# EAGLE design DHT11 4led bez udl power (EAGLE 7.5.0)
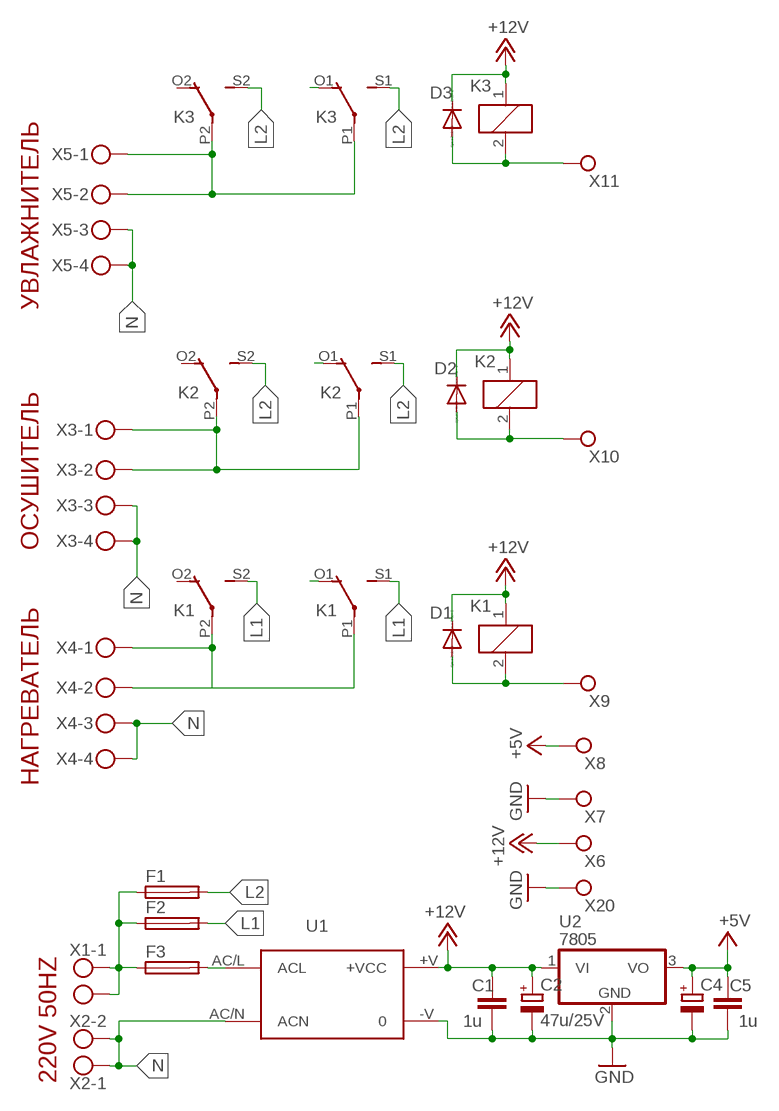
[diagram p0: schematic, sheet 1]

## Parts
C1  1u  C-EUC1206  [C1206]
C2  47u/25V  CPOL-EUE2.5-5  [E2,5-5]
C4  47u/25V  CPOL-EUE2.5-5  [E2,5-5]
C5  1u  C-EUC1206  [C1206]
D1  1N4004  [DO41-10]
D2  1N4004  [DO41-10]
D3  1N4004  [DO41-10]
F1  FUSEGSH15 10A 5x20mm  FUSEGSH15  [GSH15]
F2  FUSEGSH15 10A 5x20mm  FUSEGSH15  [GSH15]
F3  FUSEGSH15 1A 5x20mm  FUSEGSH15  [GSH15]
K1  4052  [F4052]
K2  4052  [F4052]
K3  4052  [F4052]
U1  IRM10-12  [IRM10-12]
U2  7805  7805T  [TO220H]
X1  MKDSN1,5/2-5,08  [MKDSN1,5/2-5,08]
X2  MKDSN1,5/2-5,08  [MKDSN1,5/2-5,08]
X3  MKDSN1,5/4-5,08  [MKDSN1,5/4-5,08]
X4  MKDSN1,5/4-5,08  [MKDSN1,5/4-5,08]
X5  MKDSN1,5/4-5,08  [MKDSN1,5/4-5,08]
X6  TPPAD1-17Y  [P1-17Y]
X7  TPPAD1-17Y  [P1-17Y]
X8  TPPAD1-17Y  [P1-17Y]
X9  TPPAD1-17Y  [P1-17Y]
X10  TPPAD1-17Y  [P1-17Y]
X11  TPPAD1-17Y  [P1-17Y]
X20  TPPAD1-17Y  [P1-17Y]

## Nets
+5V: C4.+ C5.1 U2.3(VO) X8.TP
+12V: C1.1 C2.+ D1.C D2.C D3.C K1.1 K2.1 K3.1 U1.+V(+VCC) U2.1(VI) X6.TP
GND: C1.2 C2.- C4.- C5.2 U1.-V U2.2(GND) X7.TP X20.TP
L1: F2.2 K1.S1(2:S) K1.S2(3:S)
L2: F1.2 K2.S1(2:S) K2.S2(3:S) K3.S1(2:S) K3.S2(3:S)
N: U1.AC/N(ACN) X2.1 X2.2 X3.3 X3.4 X4.3 X4.4 X5.3 X5.4
N$1: D3.A K3.2 X11.TP
N$2: K3.P1(2:P) K3.P2(3:P) X5.1 X5.2
N$3: K3.O1(2:O)
N$28: F1.1 F2.1 F3.1 X1.1 X1.2
N$29: F3.2 U1.AC/L(ACL)
N$41: D2.A K2.2 X10.TP
N$43: K2.P1(2:P) K2.P2(3:P) X3.1 X3.2
N$45: K2.O1(2:O)
N$48: D1.A K1.2 X9.TP
N$52: K1.O1(2:O)
N$53: K1.P1(2:P) K1.P2(3:P) X4.1 X4.2
Unconnected: K1.O2(3:O) K2.O2(3:O) K3.O2(3:O)

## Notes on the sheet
- УВЛАЖНИТЕЛЬ
- ОСУШИТЕЛЬ
- НАГРЕВАТЕЛЬ
- 220V 50HZ

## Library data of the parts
C1 C5 = rcl:C-EU: CAPACITOR, European symbol
C2 C4 = rcl:CPOL-EU: POLARIZED CAPACITOR, European symbol
D1-D3 = diode:1N4004: DIODE
F1-F3 = fuse:FUSE: Fuse; OC_FARNELL: unknown; OC_NEWARK: unknown
K1-K3 = relay:4052: RELAY 2 x switch, Finder; OC_FARNELL: unknown; OC_NEWARK: unknown
U1 = acdc:IRM10-12
U2 = linear:78*: Positive VOLTAGE REGULATOR Source: http://cache.national.com/ds/LM/LM78L05.pdf http://www.fairchildsemi.com/ds/LM/LM7805.pdf
X1 X2 = con-phoenix-508:MKDSN1,5/2-5,08: MKDSN 1,5/ 2-5,08 Printklemme
X3-X5 = con-phoenix-508:MKDSN1,5/4-5,08: MKDSN 1,5/ 4-5,08 Printklemme Nennstrom: 13,5 A Nennspannung: 250 V Rastermaß: 5,08 mm Polzahl: 4 Anschlussart: Schraubanschluss Montage: Löten Anschlussrichtung Leiter/Platine: 0 ° Artikelnummer: 1729144 Source: http://eshop.phoenixcontact.com .. 1729144.pdf
X6-X11 X20 = testpad:TP: Test pad

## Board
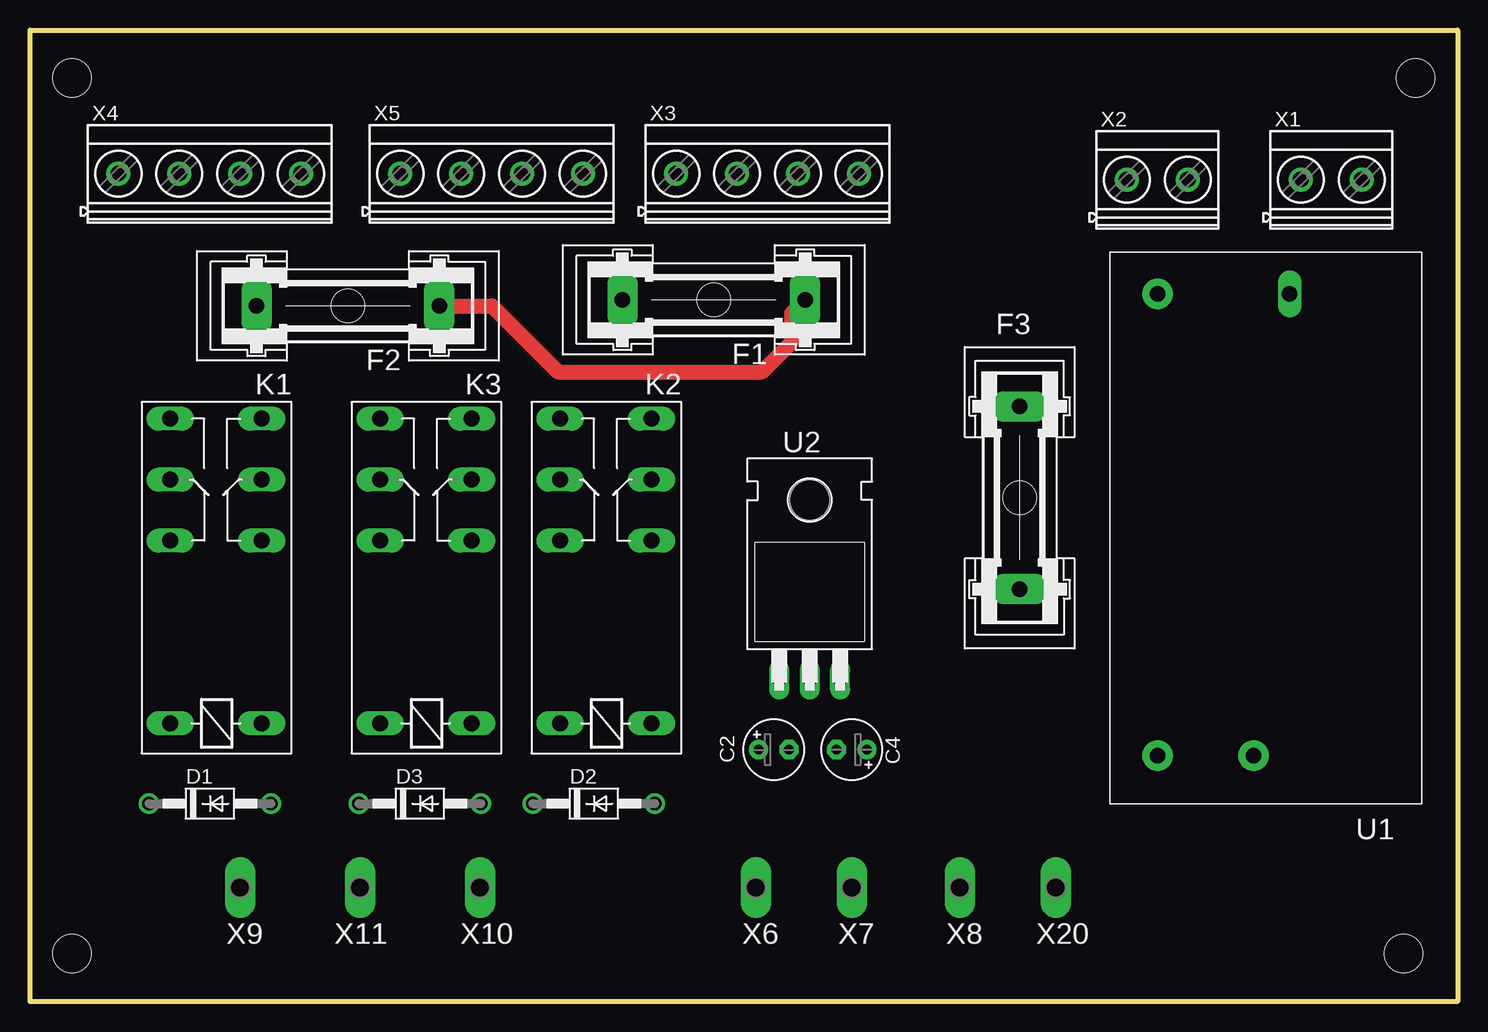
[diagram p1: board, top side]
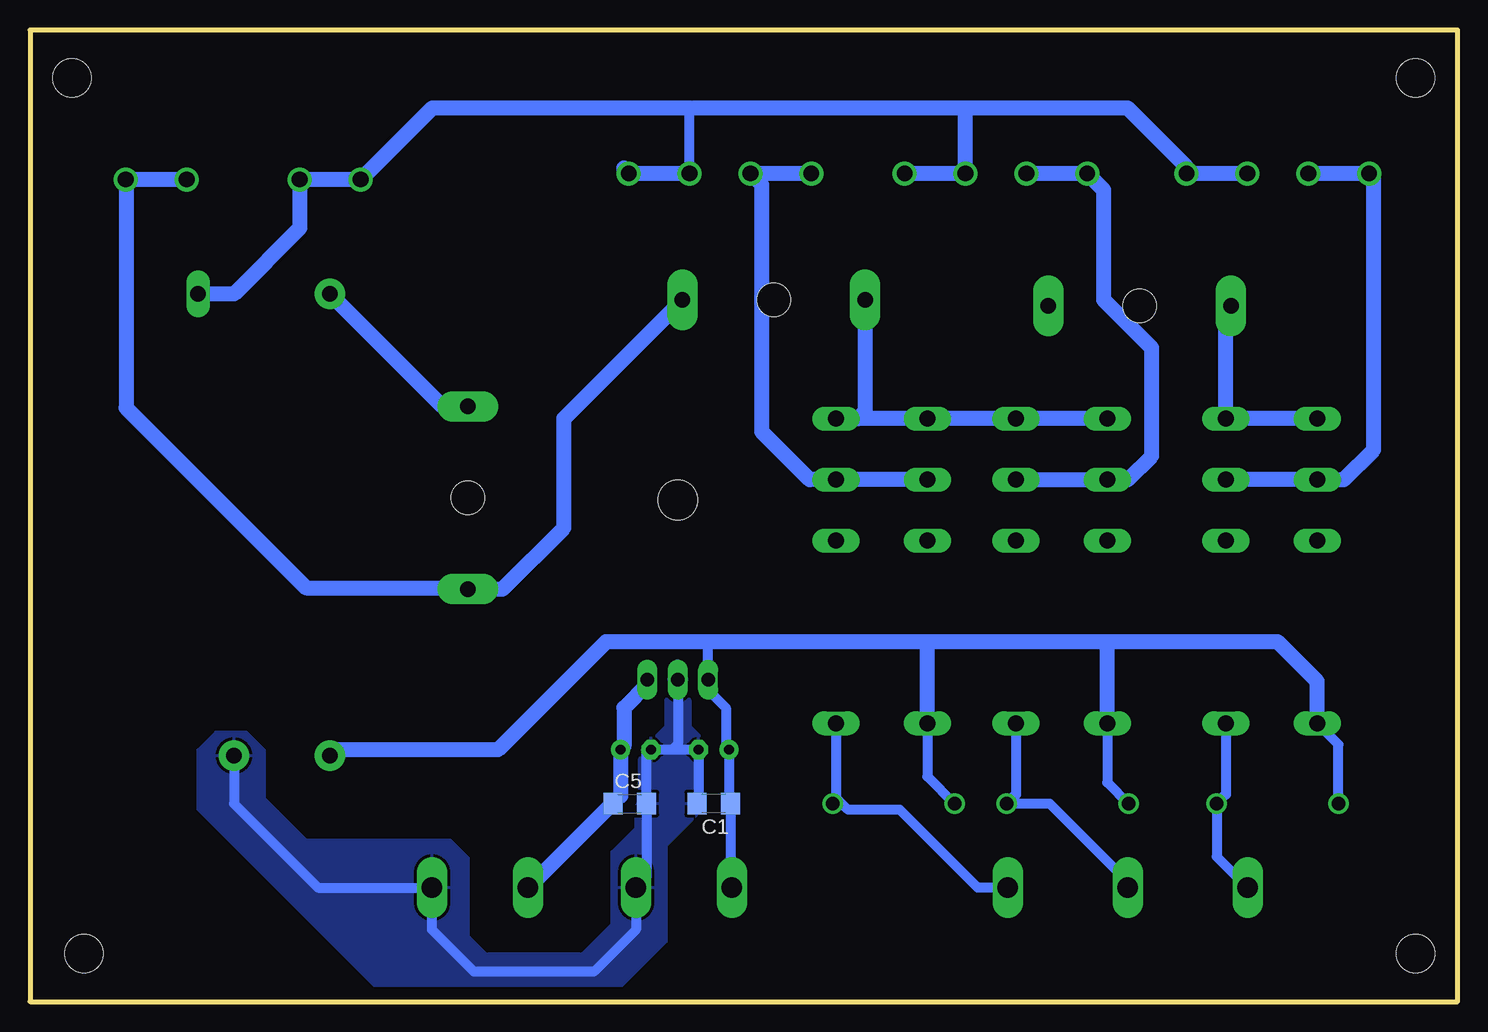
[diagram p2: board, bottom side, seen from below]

Size 119 x 81 mm. Coordinates in mm from the lower left corner, seen from the top.
Outline: 0,0 0,81 119,81 119,0 0,0
Copper layers (1*16): Top 0.035mm / dielectric 1.5mm / Bottom 0.035mm
Design rules "default": minimum track width 10mil, minimum drill 24mil, track to track 8mil, track to pad 8mil, pad to pad 8mil, via to via 8mil, smd to smd 8mil, copper to edge 40mil, drill to drill 8mil, minimum pad ring 10mil, minimum via ring 8mil, stop-mask expansion 4mil, vias tented up to drill 0mil, thermal gap 10mil
Holes 3.2 mm at -59.5,-8 3.5,77 115.5,77 205.5,-83 3.5,4 114.5,4

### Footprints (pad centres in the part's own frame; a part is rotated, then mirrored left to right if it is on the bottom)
C1206 = smd 1.6 x 1.8: 1 -1.4,0; 2 1.4,0
E2,5-5 = drill 0.813 pad 1.6: + -1.27,0 | drill 0.813 pad 1.6 octagon: - 1.27,0
DO41-10 = drill 1.118: A 5.08,0; C -5.08,0
GSH15 = drill 1.321 pad 2.54 long: 1 -7.62,0; 2 7.62,0 | hole 2.794: 0,0
F4052 = drill 1.321 long: 1 -3.81,3.81; 2 -3.81,-3.81; O1 11.43,-3.81; O2 11.43,3.81; P1 16.51,-3.81; P2 16.51,3.81; S1 21.59,-3.81; S2 21.59,3.81
IRM10-12 = drill 1.3 pad 2.54: +V 38.5,0; -V 38.5,8; AC/L 0,0 | drill 1.3 long: AC/N 0,11
TO220H = drill 1.118 long: 1 -2.54,-10.16; 2 0,-10.16; 3 2.54,-10.16 | hole 3.302: 0,4.826
MKDSN1,5/2-5,08 = drill 1.3 pad 2: 1 -2.561,0.025; 2 2.519,0.025
MKDSN1,5/4-5,08 = drill 1.3 pad 2: 1 -7.641,0.025; 2 -2.561,0.025; 3 2.519,0.025; 4 7.599,0.025
P1-17Y = drill 1.702 pad 2.121 long: TP 0,0

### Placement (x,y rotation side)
C1  62,16.5 180 bottom
C2  62,21 0 top
C4  68.5,21 180 top
C5  69,16.5 0 bottom
D1  15,16.5 0 top
D2  47,16.5 0 top
D3  32.5,16.5 0 top
F1  57,58.5 180 top
F2  26.5,58 180 top
F3  82.5,42 90 top
K1  15.5,27 90 top
K2  48,27 90 top
K3  33,27 90 top
U1  94,59 270 top
U2  65,37 0 top
X1  108.5,68.5 0 top
X2  94,68.5 0 top
X3  61.5,69 0 top
X4  15,69 0 top
X5  38.5,69 0 top
X6  60.5,9.5 0 top
X7  68.5,9.5 0 top
X8  77.5,9.5 0 top
X9  17.5,9.5 0 top
X10  37.5,9.5 0 top
X11  27.5,9.5 0 top
X20  85.5,9.5 0 top

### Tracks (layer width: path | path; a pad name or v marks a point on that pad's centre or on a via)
+5V
  Bottom 0.813: U2.3 67.54,26.46 | 69.5,21.27 C4.+ | 69.77,17.13 C5.1 70.5,16.5
  Bottom 1.27: 67.54,26.46 69.5,24.5 69.5,21.27 | C4.+ 69.77,17.13 | 70.5,16.5 X8.TP
+12V
  Bottom 0.813: X6.TP 60.6,9.6 C1.1 60.73,16.63 C2.+ 61,21.27 61,24.5 62.46,25.96 U2.1 62.5,26.88 62.5,30 | 93.5,21 U1.+V | 29.19,29.69 29.5,30 | 44.19,29.69 44.5,30 | D1.C 9.92,21.42 K1.1 | K3.1 29.19,18.27 D3.C | K2.1 44.19,18.77 D2.C
  Bottom 1.27: K1.1 11.69,26.69 15,30 29.5,30 44.5,30 62.5,30 71,30 80,21 93.5,21 | K3.1 29.19,29.69 | K2.1 44.19,29.69
GND
  Bottom 0.813: C1.2 63.27,16.63 C2.- 65.5,21 | 65.5,21 C4.- 67.6,20.63 C5.2 67.6,10.4 X7.TP 68.5,6 72,2.5 82,2.5 85.5,6 X20.TP 95,9.5 102,16.5 U1.-V | U2.2 65,21.5 65.5,21
  pour Bottom (isolate 0.813): 64,28 64,23 63,22 63,16 66,13 66,5 70.5,0.5 89.5,0.5 105,16 105,21 103.5,22.5 101,22.5 99.5,21 99.5,17 96,13.5 84,13.5 82.5,12 82.5,5.5 81,4 73,4 70.5,6.5 70.5,12.5 68.5,14.5 68.5,21 67.5,22 67,22 66,23 66,28 65.5,28.5 64.5,28.5
L1
  Bottom 1.27: K1.S2 K1.S1 19.31,57.19 19,57.5 19,57.88 F2.2
L2
  Bottom 1.27: K3.S2 K3.S1 K2.S2 50,48.59 | 50,48.59 K2.S1 | F1.2 49.38,49.21 50,48.59
N
  Bottom 0.813: 63.62,74.5 64,74.5 64.02,74.48 X3.3
  Bottom 1.27: X4.3 X4.4 22.6,69.6 27.5,74.5 41,74.5 | 41,74.5 63.62,74.5 | X3.3 69.03,69.03 69.5,69.5 69.5,69.43 X3.4 | X5.4 X5.3 41.02,74.48 41,74.5 | 64,74.5 85.46,74.5 X2.1 X2.2 96.52,64.48 102,59 U1.AC/N
N$1
  Bottom 0.813: K3.2 36.81,17.27 D3.A 34,16.5 27.5,10 X11.TP
N$2
  Bottom 1.27: K3.P2 K3.P1 27.49,43.51 25.5,45.5 25.5,54.5 29.5,58.5 29.5,67.67 X5.1 X5.2
N$28
  Top 1.27: F2.1 38.5,58 44,52.5 61,52.5 63.5,55 63.5,57.38 F1.1
  Bottom 1.27: F3.1 82,34.38 | 82,34.38 79.62,34.38 74.5,39.5 74.5,48.62 F1.1 | X1.2 X1.1 110.97,68.53 111,68.5 111,49.5 96,34.5 82.12,34.5 82,34.38
N$29
  Bottom 1.27: F3.2 84.62,49.62 U1.AC/L
N$41
  Bottom 0.813: K2.2 51.81,17 | 51.81,17 51.81,16.77 D2.A | X10.TP 40,9.5 46.5,16 50.81,16 51.81,17
N$43
  Bottom 1.27: 58.46,68.54 58,68.09 58,47.5 54.01,43.51 K2.P1 K2.P2 | 58.46,68.54 X3.2 | X3.1 57.98,69.03 58.46,68.54
N$48
  Bottom 0.813: K1.2 19.31,17.27 D1.A 20.08,12.08 X9.TP
N$53
  Bottom 1.27: X4.2 X4.1 7,68.67 7,46 9.49,43.51 K1.P2 K1.P1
